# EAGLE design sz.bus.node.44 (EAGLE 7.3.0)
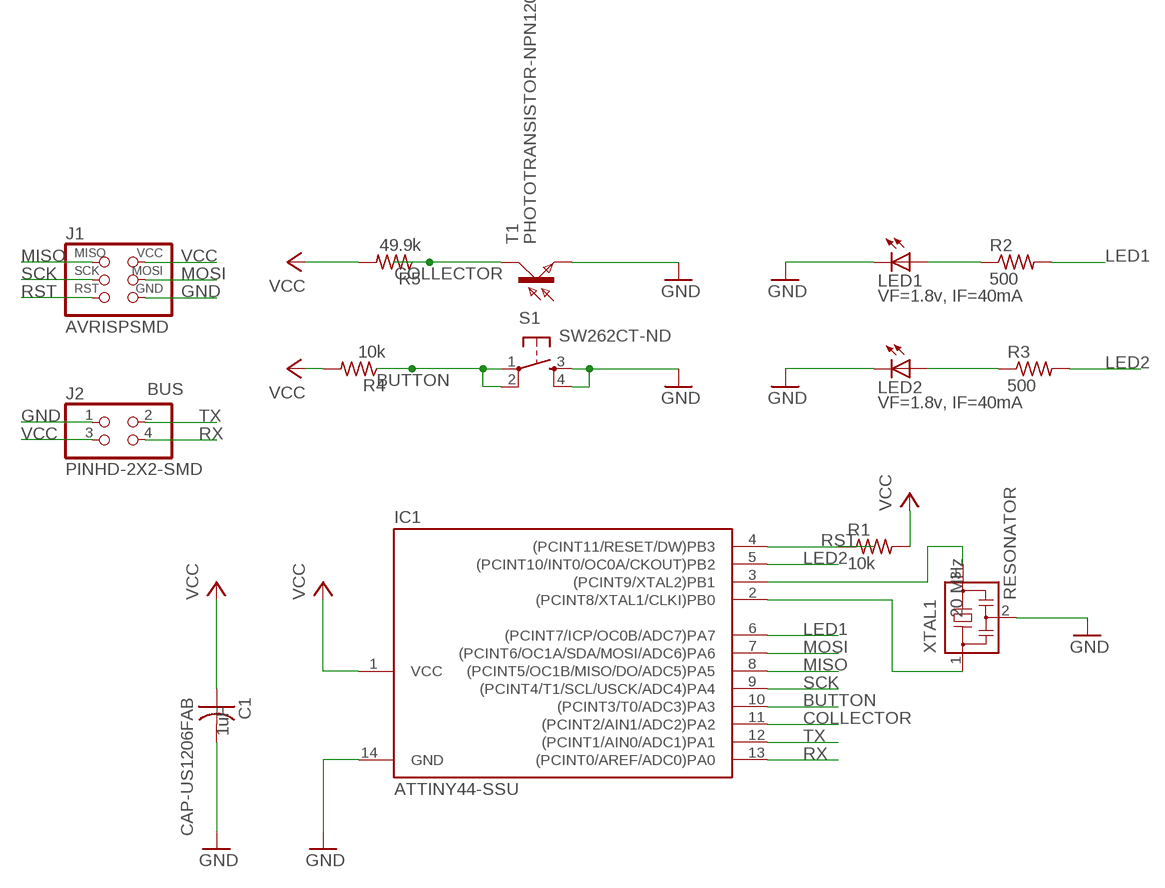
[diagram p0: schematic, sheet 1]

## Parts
C1  CAP-US1206FAB  [C1206FAB]
IC1  ATTINY44-SSU  [SOIC14]
J1  AVRISPSMD  [2X03SMD]
J2  PINHD-2X2-SMD  [2X02SMD]
LED1  VF=1.8v, IF=40mA  LEDSMT1206  [1206]
LED2  VF=1.8v, IF=40mA  LEDSMT1206  [1206]
R1  10k  RES-US1206FAB  [R1206FAB]
R2  500  RES-US1206FAB  [R1206FAB]
R3  500  RES-US1206FAB  [R1206FAB]
R4  10k  RES-US1206FAB  [R1206FAB]
R5  49.9k  RES-US1206FAB  [R1206FAB]
S1  SW262CT-ND  6MM_SWITCH6MM_SWITCH  [6MM_SWITCH]
T1  PHOTOTRANSISTOR-NPN1206  [OP1206]
XTAL1  RESONATOR  [EFOBM]

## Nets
BUTTON: IC1.10((PCINT3/T0/ADC3)PA3) R4.1 S1.1(P) S1.2(P1)
COLLECTOR: IC1.11((PCINT2/AIN1/ADC2)PA2) R5.1 T1.COLLECTOR(C)
GND: C1.2 IC1.14(GND) J1.6(GND) J2.1 LED1.C LED2.C S1.3(S) S1.4(S1) T1.EMITTER(E) XTAL1.2
LED1: IC1.6((PCINT7/ICP/OC0B/ADC7)PA7) R2.2
LED2: IC1.5((PCINT10/INT0/OC0A/CKOUT)PB2) R3.2
MISO: IC1.8((PCINT5/OC1B/MISO/DO/ADC5)PA5) J1.1(MISO)
MOSI: IC1.7((PCINT6/OC1A/SDA/MOSI/ADC6)PA6) J1.4(MOSI)
N$1: IC1.2((PCINT8/XTAL1/CLKI)PB0) XTAL1.1
N$2: LED1.A R2.1
N$3: IC1.3((PCINT9/XTAL2)PB1) XTAL1.3
N$6: LED2.A R3.1
RST: IC1.4((PCINT11/RESET/DW)PB3) J1.5(RST) R1.1
RX: IC1.13((PCINT0/AREF/ADC0)PA0) J2.4
SCK: IC1.9((PCINT4/T1/SCL/USCK/ADC4)PA4) J1.3(SCK)
TX: IC1.12((PCINT1/AIN0/ADC1)PA1) J2.2
VCC: C1.1 IC1.1(VCC) J1.2(VCC) J2.3 R1.2 R4.2 R5.2

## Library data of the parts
C1 = fab:CAP-US; CAP: 1uF
IC1 = fab:ATTINY44
J1 = fab:AVRISP
J2 = fab:PINHD-2X2-SMD
LED1 LED2 = led:LED: LED
R1-R5 = fab:RES-US: Resistor (US Symbol)
S1 = fab:6MM_SWITCH: OMRON SWITCH
T1 = fab:PHOTOTRANSISTOR-NPN
XTAL1 = fab:RESONATOR; FREQ: 20 MHz

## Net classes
0 default: width 0.305 mm, drill 0.406 mm, clearance 0.432 mm

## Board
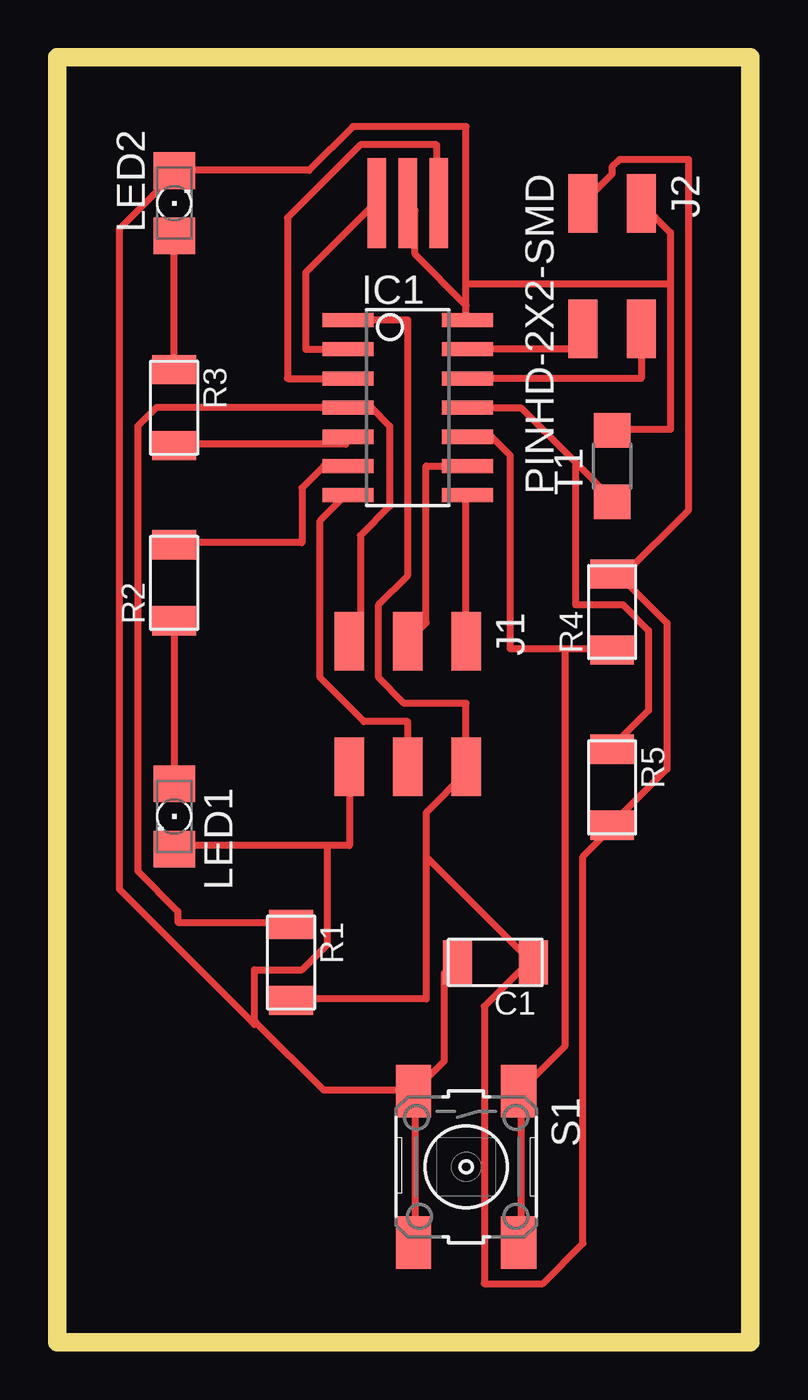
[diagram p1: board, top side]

Size 30.15 x 55.87 mm. Coordinates in mm from the lower left corner, seen from the top.
Outline: 0,0 30.15,0 30.15,55.87 0,55.87 0,0
Copper layers (1*16): Top 0.035mm / dielectric 1.5mm / Bottom 0.035mm
Design rules "default *": minimum track width 12mil, minimum drill 24mil, track to track 17mil, track to pad 17mil, pad to pad 8mil, via to via 8mil, smd to smd 8mil, copper to edge 40mil, drill to drill 8mil, minimum pad ring 10mil, minimum via ring 8mil, stop-mask expansion 4mil, vias tented up to drill 0mil, thermal gap 10mil

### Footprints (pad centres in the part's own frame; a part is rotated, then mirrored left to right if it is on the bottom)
C1206FAB = smd 1.27 x 1.905: 1 -1.651,0; 2 1.651,0
SOIC14 = smd 0.61 x 2.21: 1 -3.81,-2.603; 2 -2.54,-2.603; 3 -1.27,-2.603; 4 0,-2.603; 5 1.27,-2.603; 6 2.54,-2.603; 7 3.81,-2.603; 8 3.81,2.603; 9 2.54,2.603; 10 1.27,2.603; 11 0,2.603; 12 -1.27,2.603; 13 -2.54,2.603; 14 -3.81,2.603
2X03SMD = smd 2.54 x 1.27: 1 -2.54,2.54; 2 2.92,2.54; 3 -2.54,0; 4 2.92,0; 5 -2.54,-2.54; 6 2.92,-2.54
2X02SMD = smd 2.54 x 1.27: 1 -2.54,1.27; 2 2.92,1.27; 3 -2.54,-1.27; 4 2.92,-1.27
1206 = smd 1.6 x 1.803: A -1.422,0; C 1.422,0
R1206FAB = smd 1.27 x 1.905: 1 -1.651,0; 2 1.651,0
6MM_SWITCH = smd 2.286 x 1.524: 1 -3.302,2.286; 2 3.302,2.286; 3 -3.302,-2.286; 4 3.302,-2.286
OP1206 = smd 1.5 x 1.6: COLLECTOR -1.55,0; EMITTER 1.55,0
EFOBM = smd 0.8 x 3.9: 1 -1.35,0; 2 0,0; 3 1.35,0

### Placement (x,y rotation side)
C1  19.05,16.51 180 top
IC1  15.24,40.64 270 top
J1  15.24,27.94 270 top
J2  24.13,46.99 270 top
LED1  5.08,22.86 270 top
LED2  5.08,49.53 90 top
R1  10.16,16.51 270 top
R2  5.08,33.02 90 top
R3  5.08,40.64 270 top
R4  24.13,31.75 90 top
R5  24.13,24.13 270 top
S1  17.78,7.62 270 top
T1  24.13,38.1 90 top
XTAL1  15.24,49.53 0 top

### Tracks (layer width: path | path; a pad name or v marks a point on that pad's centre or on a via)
BUTTON
  Top 0.305: S1.2 20.16,4.45 20.16,10.79 S1.1 20.16,10.95 22.07,12.86 22.07,30.16 | 22.07,30.16 19.68,30.16 19.68,38.58 18.89,39.37 IC1.10 | 22.07,30.16 24.13,30.16 R4.1
COLLECTOR
  Top 0.305: 22.62,38.18 20.16,40.64 IC1.11 | 22.62,38.18 24.13,36.67 T1.COLLECTOR | R5.1 24.13,25.88 25.72,27.46 25.72,30.96 24.61,32.07 22.54,32.07 22.54,38.1 22.62,38.18
GND
  Top 0.305: 26.67,46.04 26.67,48.26 J2.1 | 26.67,46.04 26.67,39.69 24.13,39.69 T1.EMITTER | 17.78,45.08 17.78,44.45 IC1.14 | 17.78,45.08 17.78,46.04 | 17.78,46.04 17.78,52.86 12.86,52.86 10.95,50.96 LED2.C 5.08,50.8 2.7,48.42 2.7,19.68 8.57,13.81 8.65,13.89 | XTAL1.2 15.56,49.21 15.56,47.31 17.78,45.08 | 17.78,46.04 26.67,46.04 | 11.75,21.59 12.7,21.59 J1.6 | 11.75,21.59 5.08,21.59 LED1.C | C1.2 17.3,16.51 16.83,16.03 16.83,12.22 15.56,10.95 S1.3 | S1.4 15.56,4.45 15.56,10.79 S1.3 | 11.75,21.59 11.75,17.3 10.64,16.19 8.57,16.19 8.57,13.97 8.65,13.89 | 8.65,13.89 11.59,10.95 15.4,10.95 S1.3
LED1
  Top 0.305: IC1.6 11.59,38.1 10.64,37.15 10.64,34.77 5.08,34.77 R2.2
LED2
  Top 0.305: R3.2 5.08,39.05 12.54,39.05 12.54,39.37 IC1.5
MISO
  Top 0.305: J1.1 17.78,36.83 IC1.8
MOSI
  Top 0.305: J1.4 15.24,26.99 13.33,26.99 11.43,28.89 11.43,35.72 12.54,36.83 IC1.7
N$1
  Top 0.305: IC1.2 10.79,43.18 10.79,46.51 13.81,49.53 XTAL1.1
N$2
  Top 0.305: R2.1 LED1.A
N$3
  Top 0.305: IC1.3 10,41.91 10,48.89 13.18,52.07 16.51,52.07 16.51,49.53 XTAL1.3
N$6
  Top 0.305: R3.1 LED2.A
RST
  Top 0.305: R1.1 10.16,18.26 5.24,18.26 5.24,18.73 3.49,20.48 3.49,39.85 4.29,40.64 IC1.4 13.65,40.64 14.45,39.85 14.45,36.35 13.18,35.08 13.18,30.96 J1.5
RX
  Top 0.305: IC1.13 22.86,43.18 J2.4
SCK
  Top 0.305: IC1.9 16.03,38.1 16.03,31.27 J1.3
TX
  Top 0.305: IC1.12 25.4,41.91 J2.2
VCC
  Top 0.305: J2.3 24.13,50.8 24.13,51.12 24.45,51.43 27.46,51.43 27.46,36.2 24.61,33.34 R4.2 24.13,33.34 24.45,33.34 26.51,31.27 26.51,24.92 24.13,22.54 R5.2 24.13,22.38 22.86,21.11 22.86,4.29 21.11,2.54 18.57,2.54 18.57,14.61 20.48,16.51 C1.1 20.64,16.51 16.03,21.11 | 16.03,21.11 16.03,23.02 17.78,24.77 J1.2 17.78,27.78 15.08,27.78 13.97,28.89 13.97,32.07 15.24,33.34 15.24,44.45 IC1.1 | 16.03,21.11 16.03,14.92 10.16,14.92 R1.2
